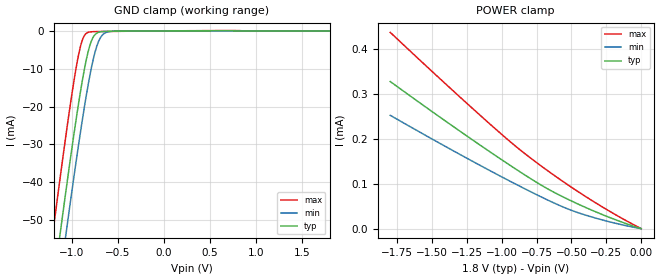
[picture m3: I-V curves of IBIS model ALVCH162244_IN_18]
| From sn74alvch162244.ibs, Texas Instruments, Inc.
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[Model]   ALVCH162244_IN_18
Model_type  Input
Vinl=0.5775
Vinh=1.2675
| variable   typ   min   max
C_comp   5.29pF   4.52pF   6.29pF
[Temperature Range]   40   100   -40
| Ambient temperature   25   85   -40
[Voltage range]   1.8   1.65   1.95
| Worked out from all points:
|   GND clamp passes 1 mA (typ) near -0.75 V on its own axis
[GND Clamp]
| ALVCH162244_IN_18
|   Voltage   I(typ)   I(min)   I(max)
-1.8V     -181.8mA   -192.8mA   -167.8mA
-1.205V   -67.7mA    -79.22mA   -52.94mA
-1.125V   -53.01mA   -64.52mA   -38.23mA
-1.06V    -41.36mA   -52.82mA   -26.69mA
-930mV    -19.52mA   -30.44mA   -6.594mA
-885mV    -12.87mA   -23.24mA   -2.306mA
-840mV    -7.2mA     -16.52mA   -586.2uA
-785mV    -2.471mA   -9.365mA   -226.7uA
-725mV    -521.7uA   -3.71mA    -179.8uA
-675mV    -184.6uA   -1.265mA   -163.2uA
-605mV    -103uA     -240.2uA   -142.7uA
1.8V      4.868pA    9.514uA    -22.72uA
[POWER Clamp]
| ALVCH162244_IN_18
|   Voltage   I(typ)   I(min)   I(max)
-1.8V     327.9uA    252.6uA    437.4uA
-1.19V    193.6uA    146.8uA    262.4uA
-970mV    147.2uA    110.5uA    201.9uA
-835mV    119.7uA    88.9uA     167.4uA
-655mV    85.98uA    61.49uA    125.6uA
-460mV    55.85uA    36.36uA    83.97uA
-235mV    25.96uA    15.89uA    40.3uA
-16.28fV  4.868pA    8.756pA    4.988pA
